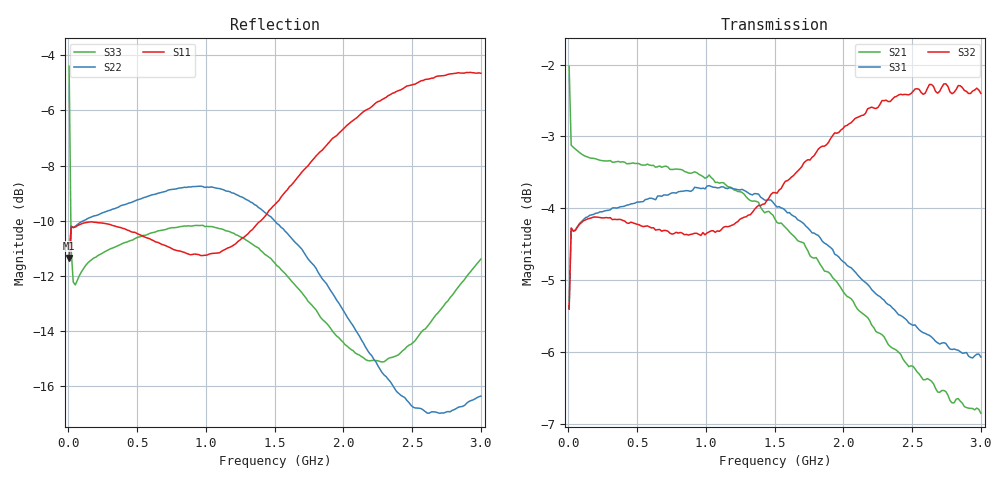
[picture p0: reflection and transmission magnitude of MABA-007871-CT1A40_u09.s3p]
#	MHz	S	RI	R	50
!FREQ	R1	I1	R2	I2	R3	I3
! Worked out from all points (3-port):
!   201 points, 5 MHz to 3 GHz, reference 50 ohm
!   strongest paths, dB at 5 MHz, 753.8 MHz, 1.502 GHz, 2.251 GHz, 3 GHz:
!     S32: -5.4, -4.4, -3.8, -2.6, -2.4
!     S31: -5.4, -3.8, -4.0, -5.2, -6.1
!     S21: -2.0, -3.5, -4.2, -5.7, -6.9
!   lowest |S11| = -11.3 dB at 5 MHz (marker M1), VSWR 1.74, Z = 74.6 + j24 ohm
!   |S11| at or under -10 dB: start of sweep to 1.399 GHz
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5  0.2262 0.1489  0.7756 -0.1551  -0.4508 -0.2921
   0.7767 -0.156  0.2233 0.1515  0.4492 0.2942
   -0.4508 -0.2921  0.4451 0.2999  -0.1017 0.5945
19.975  0.3065 0.0344  0.6951 -0.0595  -0.6066 -0.0734
        0.6956 -0.0595  0.3061 0.0449  0.6053 0.0838
        -0.6066 -0.0734  0.6056 0.0831  0.2165 0.1778
79.875  0.3102 -0.0232  0.6856 -0.0781  -0.6152 0.0228
        0.6856 -0.0772  0.3129 0.0173  0.6143 0.0186
        -0.6152 0.0228  0.6145 0.0191  0.2412 0.0713
843.6  -0.00876 -0.277  0.3869 -0.5511  -0.3771 0.5278
       0.3888 -0.5448  0.3559 -0.0753  0.5977 -0.1026
       -0.3771 0.5278  0.5957 -0.1043  0.3084 -0.0253
1173.05  -0.2189 -0.1794  0.1317 -0.6407  -0.1458 0.6358
         0.144 -0.6367  0.3273 -0.1431  0.6031 -0.1271
         -0.1458 0.6358  0.5997 -0.1271  0.2938 -0.0707
1502.5  -0.335 0.0492  -0.1368 -0.5976  0.1055 0.6255
        -0.1245 -0.6075  0.256 -0.1847  0.6284 -0.1659
        0.1055 0.6255  0.6249 -0.1674  0.2464 -0.0971
1816.975  -0.291 0.3007  -0.3317 -0.4577  0.2968 0.5262
          -0.3291 -0.4775  0.1819 -0.1785  0.6564 -0.237
          0.2968 0.5262  0.6534 -0.2325  0.1977 -0.0838
2251.25  -0.024 0.5196  -0.4545 -0.1983  0.4397 0.3282
         -0.4724 -0.2102  0.1229 -0.1211  0.6487 -0.3772
         0.4397 0.3282  0.6438 -0.368  0.1745 -0.0244
2595.675  0.2378 0.5188  -0.4593 -0.00639  0.4836 0.181
          -0.4794 -0.000214  0.1209 -0.0754  0.5943 -0.4917
          0.4836 0.181  0.5898 -0.4775  0.2003 0.0191
3000  0.4677 0.3522  -0.3993 0.1935  0.4968 0.0191
      -0.4014 0.2128  0.143 -0.0518  0.4745 -0.6039
      0.4968 0.0191  0.474 -0.592  0.2672 0.035
